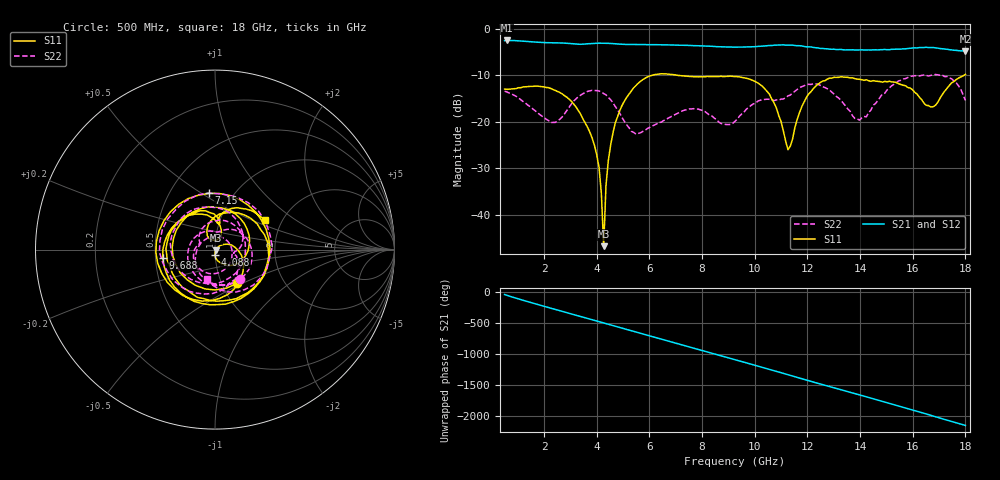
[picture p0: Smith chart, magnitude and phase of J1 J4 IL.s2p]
!Agilent Technologies,N5230A,MY45001360,A.07.50.67
!Agilent N5230A: A.07.50.67
!Date: Tuesday, April 16, 2024 16:26:41
!Correction: S11(Full 2 Port(1,2))
!S21(Full 2 Port(1,2))
!S12(Full 2 Port(1,2))
!S22(Full 2 Port(1,2))
!S2P File: Measurements: S11, S21, S12, S22:
# Hz S  dB  R 50
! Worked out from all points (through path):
!   201 points, 500 MHz to 18 GHz, reference 50 ohm
!   highest |S21| = -2.45 dB at 587.5 MHz (marker M1); lowest = -4.8 dB at 18 GHz (marker M2)
!   group delay of S21, straight-line fit = 331 ps
!   lowest |S11| = -46.8 dB at 4.263 GHz (marker M3), VSWR 1.01, Z = 50.3 - j0.306 ohm
!   |S11| at or under -10 dB: start of sweep to 6.083 GHz; 7.104 GHz to 17.94 GHz (10.83 GHz wide, 86.5 % of centre)
!   |S22| runs from -22.7 to -9.8 dB; largest |S21 - S12| = 0.0082
!   S11 on the Smith chart (normalised r, x): 500 MHz: 1.18, -0.47; 4.088 GHz: 1.00, -0.06; 7.15 GHz: 0.77, +0.54; 9.688 GHz: 0.55, -0.05; 18 GHz: 1.64, +0.60
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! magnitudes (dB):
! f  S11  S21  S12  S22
! 500 MHz  -12.9  -2.5  -2.5  -13.4
! 587.5 MHz  -13.0  -2.5  -2.4  -13.6
! 2.25 GHz  -12.8  -3.0  -2.9  -20.1
! 3.475 GHz  -19.4  -3.3  -3.2  -13.9
! 4.088 GHz  -29.9  -3.0  -3.1  -13.4
! 4.175 GHz  -35.5  -3.0  -3.0  -13.6
! 4.263 GHz  -46.8  -3.0  -3.0  -13.9
! 4.35 GHz  -33.8  -3.0  -3.1  -14.2
! 4.438 GHz  -28.4  -3.1  -3.1  -14.7
! 4.7 GHz  -20.3  -3.2  -3.2  -16.7
! 5.487 GHz  -12.2  -3.3  -3.3  -22.7
! 6.362 GHz  -9.7  -3.4  -3.4  -20.1
! 7.15 GHz  -10.0  -3.5  -3.5  -17.9
! 9.25 GHz  -10.2  -3.9  -3.9  -19.9
! 9.688 GHz  -10.6  -3.8  -3.9  -17.2
! 10.56 GHz  -14.1  -3.5  -3.5  -15.2
! 11.26 GHz  -26.0  -3.5  -3.4  -14.4
! 12.22 GHz  -12.9  -4.0  -3.9  -11.8
! 13.97 GHz  -10.8  -4.5  -4.5  -19.6
! 15.11 GHz  -11.3  -4.4  -4.4  -12.7
! 16.69 GHz  -16.8  -4.0  -4.0  -10.0
! 18 GHz  -9.8  -4.8  -4.8  -15.4
